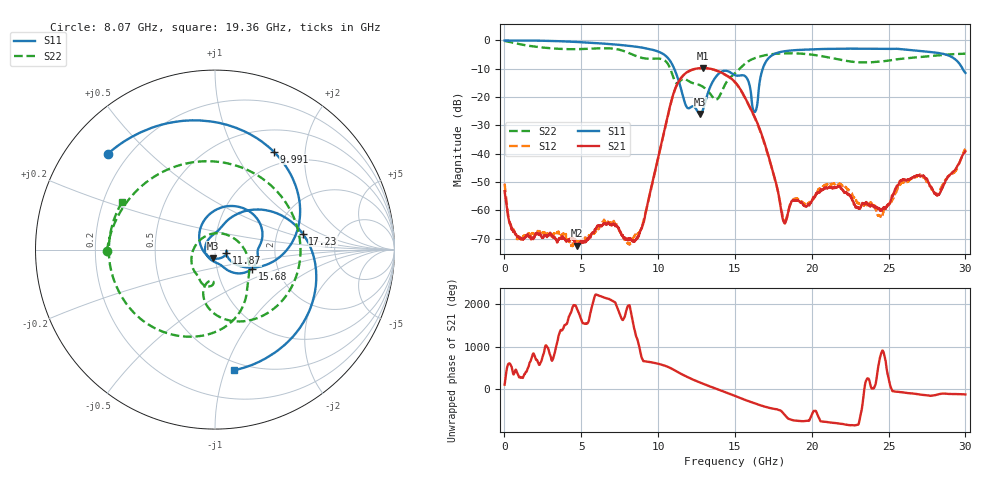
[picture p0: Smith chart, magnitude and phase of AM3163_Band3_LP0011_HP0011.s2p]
!Agilent Technologies,E8364B,MY43040894,A.07.50.67
!Agilent E8364B: A.07.50.67
!Date: Thursday, August 20, 2020 11:04:39
!Correction: S11(Full 2 Port(1,2))
!S21(Full 2 Port(1,2))
!S12(Full 2 Port(1,2))
!S22(Full 2 Port(1,2))
!S2P File: Measurements: S11, S21, S12, S22:
# Hz S  dB  R 50
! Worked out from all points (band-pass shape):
!   3201 points, 10 MHz to 30 GHz, reference 50 ohm
!   highest |S21| = -9.75 dB at 12.91 GHz (marker M1); lowest = -72.4 dB at 4.743 GHz (marker M2)
!   |S21| within 3 dB of the highest: 11.57 GHz to 14.57 GHz (3.004 GHz wide, 23 % of centre)
!   lowest |S11| = -26.0 dB at 12.73 GHz (marker M3), VSWR 1.11, Z = 48.5 - j4.71 ohm
!   |S11| at or under -10 dB: 11.05 GHz to 16.81 GHz (5.763 GHz wide, 41.4 % of centre); 29.81 GHz to end of sweep
!   |S22| runs from -20.9 to -0.3 dB; largest |S21 - S12| = 0.005
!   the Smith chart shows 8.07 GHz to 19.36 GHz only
!   S11 on the Smith chart (normalised r, x): 8.07 GHz: 0.13, +0.38; 9.991 GHz: 0.79, +1.45; 11.87 GHz: 1.13, -0.05; 15.68 GHz: 1.47, -0.33; 17.23 GHz: 2.79, +0.66; 19.36 GHz: 0.43, -1.07
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1e7  -0.05 -2.1  -53.21 111.9  -50.59 -92.4  -0.26 -6.6
9.84675e8  -0.05 -27.0  -69.94 -73.2  -69.80 -22.1  -1.36 -84.1
2.240506e9  -0.13 -61.3  -68.62 -137.1  -67.78 -64.9  -2.40 -165.8
4.742797e9  -0.59 -127.8  -72.42 68.9  -71.24 -54.5  -3.11 61.4
5.014581e9  -0.66 -135.0  -70.78 -178.3  -70.86 23.6  -3.08 46.3
6.917072e9  -1.34 173.2  -65.20 -61.3  -64.43 -64.0  -2.84 -77.8
8.069812e9  -1.93 138.1  -70.41 163.4  -71.44 -33.4  -4.40 -179.2
9.991047e9  -3.93 59.1  -41.70 -116.2  -41.92 -117.4  -6.44 -18.2
1.000979e10  -3.97 58.0  -41.24 -118.1  -41.48 -119.3  -6.45 -20.1
1.187479e10  -23.62 -18.5  -11.26 -64.0  -11.37 -63.8  -14.02 -112.4
1.272763e10  -26.02 -104.4  -9.80 161.3  -9.86 161.7  -15.83 -139.2
1.29057e10  -24.71 -156.4  -9.75 135.6  -9.80 136.0  -16.35 -148.1
1.5005e10  -12.29 2.6  -14.70 -153.6  -14.84 -153.5  -11.65 -45.5
1.567978e10  -12.72 -27.4  -20.44 110.8  -20.61 111.1  -8.15 -72.1
1.630769e10  -25.24 -177.7  -27.29 31.3  -27.56 31.8  -6.25 -99.2
1.722613e10  -6.08 10.4  -41.62 -72.0  -41.80 -68.0  -5.01 -133.7
1.819144e10  -3.86 -41.4  -64.16 141.4  -63.38 0.9  -4.59 -166.8
1.936292e10  -3.34 -81.2  -57.39 -23.9  -57.05 -27.2  -4.71 152.9
2.000958e10  -3.16 -98.9  -56.47 132.2  -56.79 -16.3  -5.04 129.0
2.25681e10  -2.94 -158.9  -55.61 -118.5  -53.55 -129.9  -7.50 13.8
2.500479e10  -3.02 145.0  -57.78 -109.7  -58.05 128.7  -7.15 -99.4
3e10  -11.50 -20.3  -39.16 -118.2  -38.26 -115.4  -4.72 100.8
